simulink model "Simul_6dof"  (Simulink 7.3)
settings: Solver=ode45  StartTime=0.0  StopTime=50  FixedStep=0.0005  MaxStep=0.015  RelTol=1e-3
InitFcn:
  | init
StartFcn:
  | init
StopFcn:
  | pl
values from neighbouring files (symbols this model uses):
  Ave = [    [vehicle_sim.m]
  Bve = [    [vehicle_sim.m]
  calfa = cos(alfa0*d2r)    [init.m]
  Cve = [    [vehicle_sim.m]
  d2r = pi/180    (= 0.0174532925199)    [init.m]    (also in robust.m)
  Dve = [    [vehicle_sim.m]
  ge = 32.174    [init.m]
  r2d = 180/pi    (= 57.2957795131)    [init.m]    (also in robust.m)
  salfa = sin(alfa0*d2r)    [init.m]
  Thet0 = 27.69    [init.m]
  V0 = 24675.1    [init.m]
undefined symbols (not defined in the file or in its folder): Kmix, Kpr, Kq

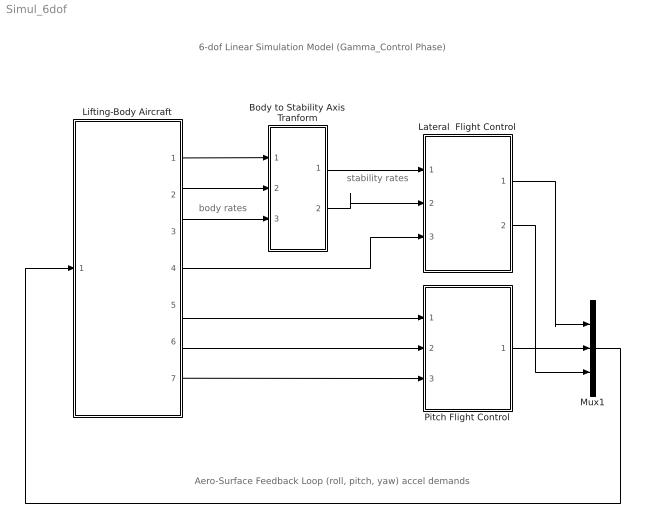
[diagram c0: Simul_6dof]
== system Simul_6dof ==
  note: 6-dof Linear Simulation Model (Gamma_Control Phase)
  note: body rates
  note: Aero-Surface Feedback Loop (roll, pitch, yaw) accel demands
  note: stability rates
  Body to Stability Axis Tranform : Subsystem
  Lateral  Flight Control : Subsystem
  Lifting-Body Aircraft : Subsystem
  Mux1 : Mux  Inputs=3
  Pitch Flight Control : Subsystem
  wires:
  Lifting-Body Aircraft/6(q) -> Pitch Flight Control/2(q)
  Lifting-Body Aircraft/7(Nz) -> Pitch Flight Control/3(Nz)
  Body to Stability Axis Tranform/2(r_s) -> Lateral  Flight Control/2(rs)
  Body to Stability Axis Tranform/1(p_s) -> Lateral  Flight Control/1(ps)
  Lifting-Body Aircraft/3(r) -> Body to Stability Axis Tranform/3(r_b)
  Lifting-Body Aircraft/2(p) -> Body to Stability Axis Tranform/2(p_b)
  Lifting-Body Aircraft/1(phi) -> Body to Stability Axis Tranform/1(phi)
  Lifting-Body Aircraft/5(gam) -> Pitch Flight Control/1(gam)
  Lifting-Body Aircraft/4(bet) -> Lateral  Flight Control/3(beta)
  Mux1/1 -> Lifting-Body Aircraft/1(PQR dem)
  Pitch Flight Control/1(dQ) -> Mux1/2
  Lateral  Flight Control/1(dP) -> Mux1/1
  Lateral  Flight Control/2(dR) -> Mux1/3

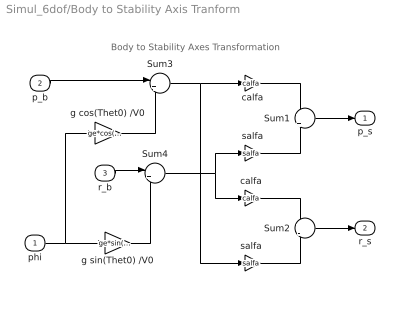
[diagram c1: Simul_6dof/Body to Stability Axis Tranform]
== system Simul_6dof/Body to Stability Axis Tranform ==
  note: Body to Stability Axes Transformation
  phi : Inport  OutDataType=sfix(16)  OutScaling=2^0
  p_b : Inport  Port=2  OutDataType=sfix(16)  OutScaling=2^0
  r_b : Inport  Port=3  OutDataType=sfix(16)  OutScaling=2^0
  Sum1 : Sum  Inputs=+|+  OutDataType=sfix(16)  OutScaling=2^0
  Sum2 : Sum  Inputs=+|-  OutDataType=sfix(16)  OutScaling=2^0
  Sum3 : Sum  Inputs=|++  OutDataType=sfix(16)  OutScaling=2^0
  Sum4 : Sum  Inputs=|+-  OutDataType=sfix(16)  OutScaling=2^0
  calfa : Gain  Gain=calfa  ParameterDataType=sfix(16)  ParameterScaling=2^0  OutDataType=sfix(16)  OutScaling=2^0
  "calfa " : Gain  Gain=calfa  ParameterDataType=sfix(16)  ParameterScaling=2^0  OutDataType=sfix(16)  OutScaling=2^0
  g cos(Thet0) /V0 : Gain  Gain=ge*cos(Thet0*d2r)/V0  ParameterDataType=sfix(16)  ParameterScaling=2^0  OutDataType=sfix(16)  OutScaling=2^0
  g sin(Thet0) /V0 : Gain  Gain=ge*sin(Thet0*d2r)/V0  ParameterDataType=sfix(16)  ParameterScaling=2^0  OutDataType=sfix(16)  OutScaling=2^0
  salfa : Gain  Gain=salfa  ParameterDataType=sfix(16)  ParameterScaling=2^0  OutDataType=sfix(16)  OutScaling=2^0
  "salfa " : Gain  Gain=salfa  ParameterDataType=sfix(16)  ParameterScaling=2^0  OutDataType=sfix(16)  OutScaling=2^0
  p_s : Outport  OutDataType=sfix(16)  OutScaling=2^0
  r_s : Outport  Port=2  OutDataType=sfix(16)  OutScaling=2^0
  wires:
  "salfa "/1 -> Sum2/2
  "calfa "/1 -> Sum2/1
  salfa/1 -> Sum1/2
  calfa/1 -> Sum1/1
  Sum3/1 -> calfa/1, "salfa "/1
  Sum4/1 -> salfa/1, "calfa "/1
  phi/1 -> g sin(Thet0) /V0/1, g cos(Thet0) /V0/1
  g sin(Thet0) /V0/1 -> Sum4/2
  g cos(Thet0) /V0/1 -> Sum3/2
  r_b/1 -> Sum4/1
  p_b/1 -> Sum3/1
  Sum2/1 -> r_s/1
  Sum1/1 -> p_s/1

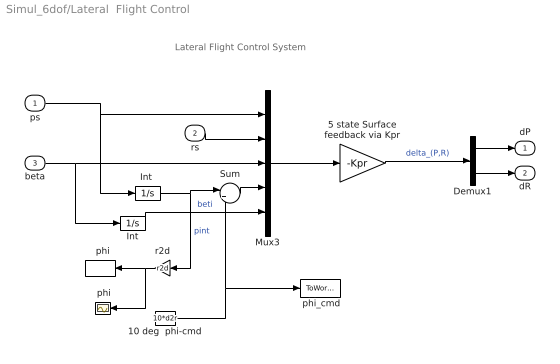
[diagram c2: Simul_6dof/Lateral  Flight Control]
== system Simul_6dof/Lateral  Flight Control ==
  note: Lateral Flight Control System
  ps : Inport  OutDataType=sfix(16)  OutScaling=2^0
  rs : Inport  Port=2  OutDataType=sfix(16)  OutScaling=2^0
  beta : Inport  Port=3  OutDataType=sfix(16)  OutScaling=2^0
  "  phi" : ToWorkspace  VariableName=phist  SampleTime=-1  SaveFormat=Array
  " phi" : Scope
  " phi_cmd" : ToWorkspace  VariableName=phicmd  SampleTime=-1  SaveFormat=Array
  10 deg  phi-cmd : Constant  Value=10*d2r  OutDataType=sfix(16)  OutScaling=2^0
  5 state Surface feedback via Kpr : Gain  Gain=-Kpr  Multiplication=Matrix(K*u)  ParameterDataType=sfix(16)  ParameterScaling=2^0  OutDataType=sfix(16)  OutScaling=2^0
  Demux1 : Demux  Outputs=2
  Int : Integrator
  "Int " : Integrator
  Mux3 : Mux  Inputs=5
  Sum : Sum  Inputs=|+-  OutDataType=sfix(16)  OutScaling=2^0
  r2d : Gain  Gain=r2d  ParameterDataType=sfix(16)  ParameterScaling=2^0  OutDataType=sfix(16)  OutScaling=2^0
  dP : Outport  OutDataType=sfix(16)  OutScaling=2^0
  dR : Outport  Port=2  OutDataType=sfix(16)  OutScaling=2^0
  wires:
  Mux3/1 -> 5 state Surface feedback via Kpr/1
  5 state Surface feedback via Kpr/1 -> Demux1/1  "delta_(P,R)"
  r2d/1 -> "  phi"/1, " phi"/1
  10 deg  phi-cmd/1 -> " phi_cmd"/1, Sum/2
  rs/1 -> Mux3/2
  ps/1 -> Mux3/1, "Int "/1
  beta/1 -> Mux3/3, Int/1
  Int/1 -> Mux3/5  "beti"
  Sum/1 -> Mux3/4
  "Int "/1 -> r2d/1, Sum/1  "pint"
  Demux1/1 -> dP/1
  Demux1/2 -> dR/1

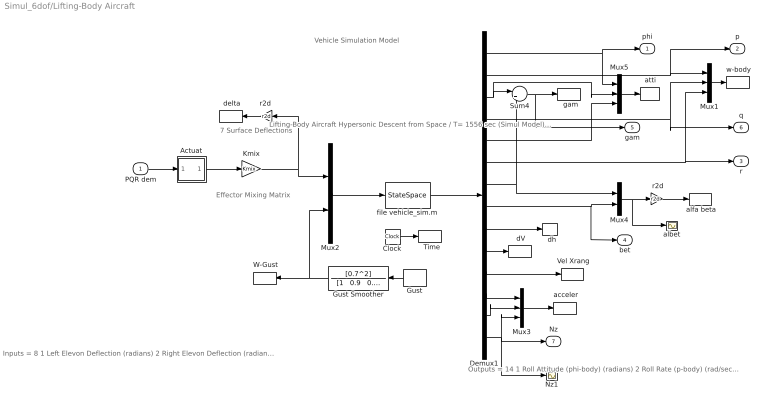
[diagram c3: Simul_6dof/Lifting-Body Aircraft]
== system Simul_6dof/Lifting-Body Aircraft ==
  note: 7 Surface Deflections
  note: Vehicle Simulation Model
  note: Outputs = 14 1 Roll Attitude (phi-body) (radians) 2 Roll Rate (p-body) (rad/sec) 3 Pitch Attitude (thet-bdy) (radians) 4 Pitch Rate (q-body) (rad/sec) 5 Yaw Attitude (psi-body) (radians) 6 Yaw Rate (r-body) (rad/sec) 7 Angle of attack, alfa, (radians) 8 Angle of sideslip, beta, (radian) 9 Change in Altitude, delta-h, (feet) 10 Forward Acceleration (V-dot) (ft/sec) 11 Cross Range Velocity (Vcr) (ft/sec) 12 CG Acceleration along X axis, (ft/sec^2) 13 CG Acceleration along Y axis, (ft/sec^2) 14 CG Acceleration along Z axis, (ft/sec^2)
  note: Effector Mixing Matrix
  note: Lifting-Body Aircraft Hypersonic Descent from Space / T= 1556 sec (Simul Model) Gamma_Control Phase
  note: Inputs = 8 1 Left Elevon Deflection (radians) 2 Right Elevon Deflection (radians) 3 Rudder Deflection (radians) 4 Upper Left Body-Flap Deflection (radians) 5 Upper Right Body-Flap Deflection (radians) 6 Lower Left Body-Flap Deflection (radians) 7 Lower Right Body-Flap Deflection (radians) 8 Wind Gust Azim, Elev Angles=(45 , 90) (deg)
  PQR dem : Inport  OutDataType=sfix(16)  OutScaling=2^0
  "  Time" : ToWorkspace  VariableName=time  SampleTime=-1  SaveFormat=Array
  "  dh" : ToWorkspace  VariableName=dh  SampleTime=-1  SaveFormat=Array
  "  gam" : ToWorkspace  VariableName=gama  SampleTime=-1  SaveFormat=Array
  " Vel Xrang" : ToWorkspace  VariableName=VXR  SampleTime=-1  SaveFormat=Array
  " W-Gust" : ToWorkspace  VariableName=gust  SampleTime=-1  SaveFormat=Array
  " acceler" : ToWorkspace  VariableName=accel  SampleTime=-1  SaveFormat=Array
  " alfa beta" : ToWorkspace  VariableName=albet  SampleTime=-1  SaveFormat=Array
  " atti" : ToWorkspace  VariableName=atti  SampleTime=-1  SaveFormat=Array
  " dV" : ToWorkspace  VariableName=dV  SampleTime=-1  SaveFormat=Array
  " delta" : ToWorkspace  VariableName=delta  SampleTime=-1  SaveFormat=Array
  " r2d" : Gain  Gain=r2d  ParameterDataType=sfix(16)  ParameterScaling=2^0  OutDataType=sfix(16)  OutScaling=2^0
  " w-body" : ToWorkspace  VariableName=pqr  SampleTime=-1  SaveFormat=Array
  Actuat : Subsystem
  Clock : Clock
  Demux1 : Demux  Outputs=14
  Gust : DiscretePulseGenerator  PulseType=Time based  Amplitude=00  Period=300  PulseWidth=2  PhaseDelay=30  SampleTime=1
  Gust Smoother : TransferFcn  Numerator=[0.7^2]  Denominator="[1   0.9   0.7^2]"
  Kmix : Gain  Gain=Kmix  Multiplication=Matrix(K*u)  ParameterDataType=sfix(16)  ParameterScaling=2^0  OutDataType=sfix(16)  OutScaling=2^0
  Mux1 : Mux  Inputs=3
  Mux2 : Mux  Inputs=[7, 1]
  Mux3 : Mux  Inputs=3
  Mux4 : Mux  Inputs=2
  Mux5 : Mux  Inputs=3
  Nz1 : Scope
  Sum4 : Sum  Inputs=|+-  OutDataType=sfix(16)  OutScaling=2^0
  albet : Scope
  file vehicle_sim.m : StateSpace  A=Ave  B=Bve  C=Cve  D=Dve
  "r2d " : Gain  Gain=r2d  ParameterDataType=sfix(16)  ParameterScaling=2^0  OutDataType=sfix(16)  OutScaling=2^0
  phi : Outport  OutDataType=sfix(16)  OutScaling=2^0
  p : Outport  Port=2  OutDataType=sfix(16)  OutScaling=2^0
  r : Outport  Port=3  OutDataType=sfix(16)  OutScaling=2^0
  bet : Outport  Port=4  OutDataType=sfix(16)  OutScaling=2^0
  gam : Outport  Port=5  OutDataType=sfix(16)  OutScaling=2^0
  q : Outport  Port=6  OutDataType=sfix(16)  OutScaling=2^0
  Nz : Outport  Port=7  OutDataType=sfix(16)  OutScaling=2^0
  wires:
  Mux2/1 -> file vehicle_sim.m/1
  Kmix/1 -> "r2d "/1, Mux2/1
  Demux1/2 -> Mux1/1, p/1
  Demux1/4 -> Mux1/2, q/1
  Demux1/6 -> Mux1/3, r/1
  Demux1/8 -> Mux4/2, bet/1
  PQR dem/1 -> Actuat/1(in)
  "r2d "/1 -> " delta"/1
  Demux1/1 -> Mux5/1, phi/1
  file vehicle_sim.m/1 -> Demux1/1
  Demux1/9 -> "  dh"/1
  Demux1/10 -> " dV"/1
  Demux1/11 -> " Vel Xrang"/1
  Gust/1 -> Gust Smoother/1
  Gust Smoother/1 -> " W-Gust"/1, Mux2/2
  Mux1/1 -> " w-body"/1
  Demux1/13 -> Mux3/2
  Demux1/12 -> Mux3/1
  Mux3/1 -> " acceler"/1
  Clock/1 -> "  Time"/1
  " r2d"/1 -> " alfa beta"/1
  Mux4/1 -> " r2d"/1, albet/1
  Demux1/3 -> Sum4/1, Mux5/2
  Sum4/1 -> "  gam"/1, gam/1
  Mux5/1 -> " atti"/1
  Demux1/5 -> Mux5/3
  Demux1/14 -> Nz/1, Mux3/3, Nz1/1
  Demux1/7 -> Sum4/2, Mux4/1
  Actuat/1(ou) -> Kmix/1

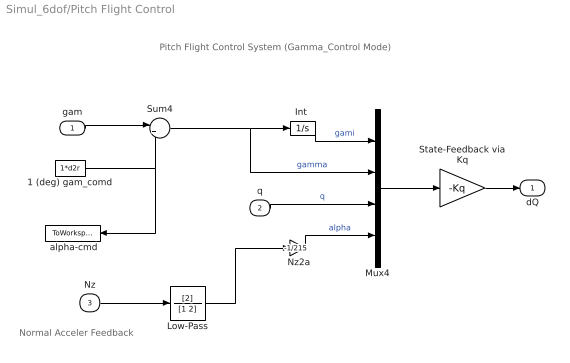
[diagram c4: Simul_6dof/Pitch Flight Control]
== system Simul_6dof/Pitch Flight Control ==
  note: Pitch Flight Control System (Gamma_Control Mode)
  note: Normal Acceler Feedback
  gam : Inport  OutDataType=sfix(16)  OutScaling=2^0
  q : Inport  Port=2  OutDataType=sfix(16)  OutScaling=2^0
  Nz : Inport  Port=3  OutDataType=sfix(16)  OutScaling=2^0
  " Nz2a" : Gain  Gain=-1/215  ParameterDataType=sfix(16)  ParameterScaling=2^0  OutDataType=sfix(16)  OutScaling=2^0
  " alpha-cmd" : ToWorkspace  VariableName=gama_cmd  SampleTime=-1  SaveFormat=Array
  1 (deg) gam_comd : Constant  Value=1*d2r  OutDataType=sfix(16)  OutScaling=2^0
  "Int " : Integrator
  Low-Pass : TransferFcn  Numerator=[2]  Denominator=[1 2]
  Mux4 : Mux
  State-Feedback via Kq : Gain  Gain=-Kq  Multiplication=Matrix(K*u)  ParameterDataType=sfix(16)  ParameterScaling=2^0  OutDataType=sfix(16)  OutScaling=2^0
  Sum4 : Sum  Inputs=|+-  OutDataType=sfix(16)  OutScaling=2^0
  dQ : Outport  OutDataType=sfix(16)  OutScaling=2^0
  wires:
  State-Feedback via Kq/1 -> dQ/1
  Mux4/1 -> State-Feedback via Kq/1
  q/1 -> Mux4/3  "q"
  "Int "/1 -> Mux4/1  "gami"
  gam/1 -> Sum4/1
  Sum4/1 -> "Int "/1, Mux4/2  "gamma"
  1 (deg) gam_comd/1 -> Sum4/2, " alpha-cmd"/1
  " Nz2a"/1 -> Mux4/4  "alpha"
  Low-Pass/1 -> " Nz2a"/1
  Nz/1 -> Low-Pass/1

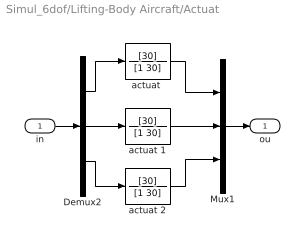
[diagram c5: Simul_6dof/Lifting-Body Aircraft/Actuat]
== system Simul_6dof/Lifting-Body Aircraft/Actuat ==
  in : Inport
  Demux2 : Demux  Outputs=3
  Mux1 : Mux  Inputs=3
  "actuat " : TransferFcn  Numerator=[30]  Denominator=[1 30]
  actuat 1 : TransferFcn  Numerator=[30]  Denominator=[1 30]
  actuat 2 : TransferFcn  Numerator=[30]  Denominator=[1 30]
  ou : Outport
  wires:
  actuat 1/1 -> Mux1/2
  "actuat "/1 -> Mux1/1
  actuat 2/1 -> Mux1/3
  Demux2/2 -> actuat 1/1
  Demux2/1 -> "actuat "/1
  Demux2/3 -> actuat 2/1
  in/1 -> Demux2/1
  Mux1/1 -> ou/1
